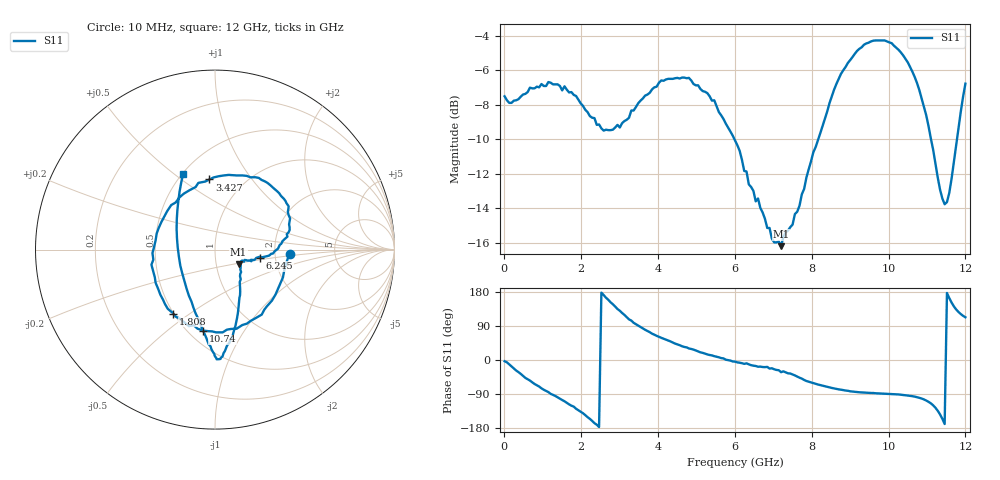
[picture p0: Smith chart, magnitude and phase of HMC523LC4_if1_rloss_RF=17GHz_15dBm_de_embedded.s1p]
!Hittite Microwave Corporation
!20 Alpha Rd
!Chelmsford, MA 01824
!Tel: 978-250-3343
!Fax: 978-250-3373
!Device: HMC523LC4, 0.01-12 GHz, GaAs MMIC Double-Balanced Mixer
!Misc: IF1 Return Loss with RF=17GHz at 15 dBm, Room
# MHZ S MA R 50
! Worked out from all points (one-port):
!   201 points, 10 MHz to 12 GHz, reference 50 ohm
!   lowest |S11| = -16.2 dB at 7.204 GHz (marker M1), VSWR 1.37, Z = 64.1 - j10.8 ohm
!   |S11| at or under -10 dB: 5.991 GHz to 8.172 GHz (2.181 GHz wide, 30.8 % of centre); 11.11 GHz to 11.78 GHz (674.4 MHz wide, 5.89 % of centre)
!   S11 on the Smith chart (normalised r, x): 10 MHz: 2.44, -0.14; 1.808 GHz: 0.50, -0.43; 3.427 GHz: 0.70, +0.64; 6.245 GHz: 1.66, -0.16; 10.74 GHz: 0.59, -0.68; 12 GHz: 0.51, +0.54
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10  0.421 -3.2
549.55  0.428 -47.2
849.3  0.449 -66.7
1149.05  0.463 -84.7
1508.75  0.438 -105.6
1808.5  0.425 -123.0
2348.05  0.364 -166.7
2707.75  0.336 158.9
3007.5  0.342 129.9
3427.15  0.392 94.5
4086.6  0.468 58.6
4506.25  0.476 41.3
4806  0.476 30.5
5285.6  0.43 14.7
6005  0.314 -4.2
6244.8  0.256 -10.2
6964.2  0.163 -21.8
7204  0.155 -32.1
7503.75  0.179 -38.0
8582.85  0.44 -75.0
9002.5  0.536 -82.6
9901.75  0.611 -89.2
10501.25  0.528 -93.8
10741.05  0.46 -98.1
11160.7  0.295 -119.6
11460.45  0.205 -168.9
11580.35  0.221 163.4
12000  0.458 112.8
